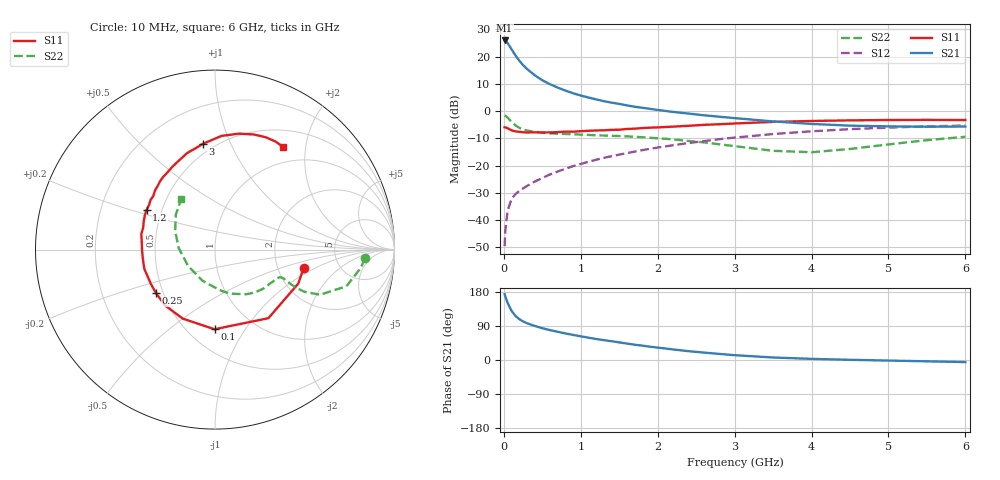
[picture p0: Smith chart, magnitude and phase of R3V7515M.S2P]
! SIEMENS Small Signal Semiconductors
! BFR181
! Si NPN RF Bipolar Junction Transistor in SOT23
! VCE = 0.75 V  IC = 15 mA
! Common Emitter S-Parameters:  May  1996
# GHz  S  MA  R  50
!  f  S11  S21  S12  S22
! GHz  MAG  ANG  MAG  ANG  MAG  ANG  MAG  ANG
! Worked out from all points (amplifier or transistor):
!   36 points, 10 MHz to 6 GHz, reference 50 ohm
!   highest |S21| = 26.0 dB at 10 MHz (marker M1)
!   |S21| within 3 dB of that: start of sweep to 94.69 MHz
!   unconditionally stable (mu >= 1): start of sweep to 19.57 MHz; 179.6 MHz to end of sweep
!   at 250 MHz: K = 1.21, MAG = 19.9 dB, |S12| = -28.4 dB
!   at 1.4 GHz: K = 1.58, MAG = 5.3 dB, |S12| = -16.6 dB
!   at 6 GHz: K = 1.20, MAG = -2.9 dB, |S12| = -5.3 dB
!   S11 on the Smith chart (normalised r, x): 10 MHz: 2.80, -0.76; 100 MHz: 0.67, -0.74; 250 MHz: 0.46, -0.27; 1.2 GHz: 0.41, +0.23; 3 GHz: 0.44, +0.79; 6 GHz: 0.74, +1.61
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0.01  0.5043 -11.5  19.88 173.6  0.0033 78.6  0.8355 -3.3
0.02  0.5013 -22.1  19.51 167.1  0.0066 78.4  0.8206 -6.9
0.05  0.4843 -52.1  17.73 150.3  0.015 69.8  0.7603 -15.6
0.1  0.4437 -90.3  13.7 129.8  0.0242 60.0  0.6358 -23.3
0.15  0.4243 -115.0  10.61 116.6  0.0298 56.3  0.5482 -25.3
0.2  0.4175 -131.6  8.486 108.0  0.0341 55.8  0.4942 -25.1
0.25  0.4086 -143.5  6.996 101.8  0.038 56.7  0.46 -24.4
0.3  0.4051 -151.8  5.968 97.1  0.0421 58.9  0.4403 -23.6
0.4  0.4081 -164.7  4.582 90.0  0.0506 61.2  0.4161 -22.8
0.5  0.4053 -173.6  3.694 83.9  0.0591 63.5  0.4002 -22.7
0.6  0.4067 179.6  3.125 78.9  0.0686 65.2  0.3909 -23.2
0.8  0.4197 168.1  2.386 70.2  0.0873 66.8  0.3809 -25.2
0.9  0.4183 163.2  2.13 66.2  0.0975 67.2  0.3757 -26.6
1.1  0.4353 153.9  1.777 58.9  0.1173 67.3  0.3653 -30.0
1.2  0.4411 149.7  1.643 55.4  0.128 67.1  0.3598 -31.8
1.7  0.4762 132.3  1.204 40.3  0.18 64.1  0.3379 -41.8
2.2  0.5192 117.2  0.967 27.9  0.2361 59.5  0.3031 -55.1
3  0.5926 96.7  0.744 12.7  0.3263 49.5  0.2273 -83.5
3.5  0.6345 86.7  0.647 6.6  0.3794 42.4  0.1866 -112.3
4.5  0.6766 71.5  0.541 0.5  0.4659 27.3  0.2018 178.0
5.5  0.6902 60.7  0.517 -3.5  0.5243 13.4  0.2927 138.2
6  0.686 56.4  0.521 -5.5  0.5445 6.5  0.3374 124.1
